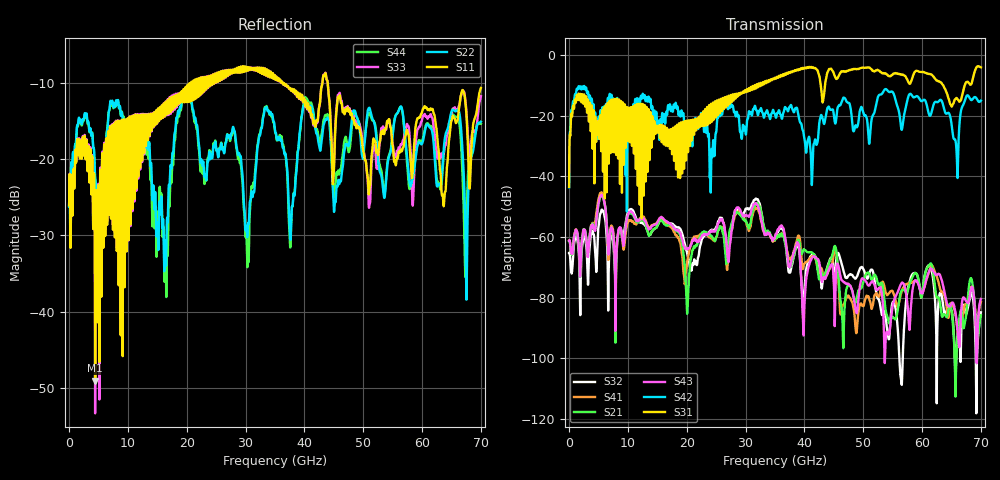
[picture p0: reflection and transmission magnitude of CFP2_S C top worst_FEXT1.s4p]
! AWR Design Environment (8415) Tue Jan 08 13:15:55 2019
! Document = 'CFP2 Channel_S'
! nPorts: 4, nXvals: 7001
# HZ S DB R 50
!Freq DBS11 AngS11 DBS12 AngS12 DBS13 AngS13 DBS14 AngS14
!	DBS21 AngS21 DBS22 AngS22 DBS23 AngS23 DBS24 AngS24
!	DBS31 AngS31 DBS32 AngS32 DBS33 AngS33 DBS34 AngS34
!	DBS41 AngS41 DBS42 AngS42 DBS43 AngS43 DBS44 AngS44
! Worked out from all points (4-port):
!   7000 points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, 10 MHz to 70 GHz, reference 50 ohm
!   strongest paths, dB at 10 MHz, 17.51 GHz, 35.01 GHz, 52.51 GHz, 70 GHz:
!     S31: -43.4, -32.7, -7.5, -5.0, -4.0
!     S42: -43.6, -17.3, -19.5, -13.8, -15.0
!     S43: -61.2, -56.2, -59.8, -77.2, -80.4
!     S21: -61.4, -56.1, -60.8, -75.2, -85.8
!     S41: -61.1, -57.1, -60.9, -79.4, -81.3
!     S32: -65.3, -55.6, -60.5, -80.3, -84.8
!   lowest |S11| = -49.0 dB at 4.43 GHz (marker M1), VSWR 1.01, Z = 49.9 + j0.337 ohm
!   |S11| at or under -10 dB: start of sweep to 20.77 GHz; 36.28 GHz to 43.07 GHz (6.792 GHz wide, 17.1 % of centre); 43.96 GHz to end of sweep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
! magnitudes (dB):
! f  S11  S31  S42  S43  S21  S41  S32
! 10 MHz  -26.1  -43.4  -43.6  -61.2  -61.4  -61.1  -65.3
! 1.36 GHz  -17.4  -13.5  -11.1  -58.2  -58.3  -58.2  -60.3
! 4.43 GHz  -49.0  -20.4  -18.9  -57.9  -57.4  -55.2  -64.7
! 20.1 GHz  -10.5  -22.7  -23.0  -64.0  -84.8  -67.8  -65.6
! 31.81 GHz  -8.4  -10.3  -18.1  -48.9  -49.0  -50.4  -47.4
! 39.86 GHz  -12.2  -4.3  -25.8  -92.4  -64.0  -69.4  -86.7
! 70 GHz  -10.7  -4.0  -15.0  -80.4  -85.8  -81.3  -84.8
